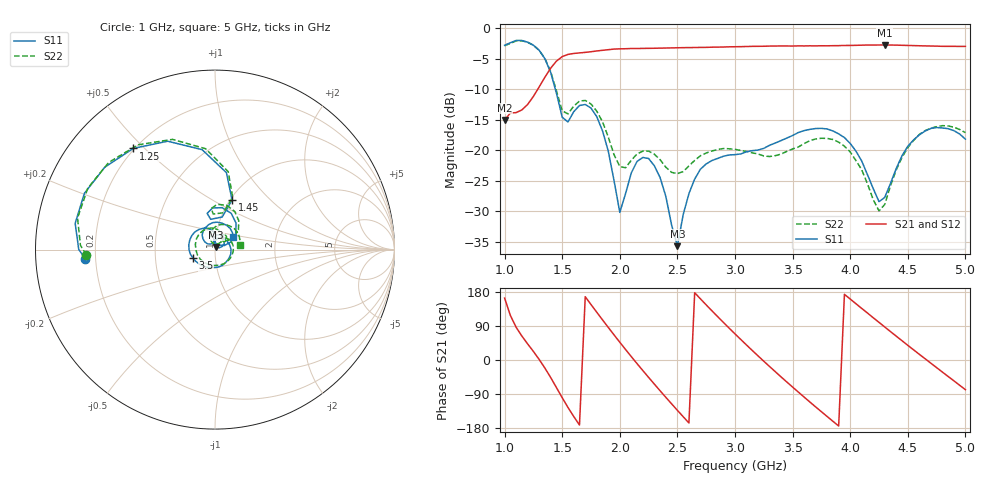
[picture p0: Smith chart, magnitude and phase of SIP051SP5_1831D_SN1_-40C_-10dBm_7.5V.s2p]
# GHz  S  dB  R  50
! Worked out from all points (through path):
!   81 points, 1 GHz to 5 GHz, reference 50 ohm
!   highest |S21| = -2.76 dB at 4.3 GHz (marker M1); lowest = -15.0 dB at 1 GHz (marker M2)
!   lowest |S11| = -35.7 dB at 2.5 GHz (marker M3), VSWR 1.03, Z = 50.6 + j1.55 ohm
!   |S11| at or under -10 dB: 1.44 GHz to end of sweep
!   |S22| runs from -29.9 to -2.1 dB; largest |S21 - S12| = 0.0026
!   S11 on the Smith chart (normalised r, x): 1 GHz: 0.16, -0.04; 1.25 GHz: 0.20, +0.46; 1.45 GHz: 1.02, +0.62; 3.5 GHz: 0.78, -0.07; 5 GHz: 1.21, +0.17
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1  -2.81 -175.9  -15.05 163.3  -15.04 163.5  -2.88 -177.6
1.15  -2.02 156.6  -13.39 63.0  -13.39 63.1  -2.08 154.2
1.25  -2.80 128.9  -11.18 22.6  -11.18 22.5  -2.80 126.3
1.45  -10.67 71.1  -5.40 -72.8  -5.39 -72.8  -10.26 71.2
1.55  -15.37 98.1  -4.30 -125.2  -4.30 -125.1  -14.05 92.8
1.7  -12.51 80.3  -3.97 167.0  -3.97 167.0  -11.85 75.3
1.9  -20.16 25.6  -3.53 86.0  -3.51 86.0  -17.85 33.5
2  -30.19 57.9  -3.39 46.9  -3.38 46.7  -22.66 46.4
2.1  -23.71 96.7  -3.34 8.9  -3.34 8.9  -21.64 66.1
2.35  -24.49 31.9  -3.28 -81.3  -3.27 -81.2  -21.56 40.2
2.5  -35.72 69.2  -3.22 -132.9  -3.22 -132.8  -23.84 47.2
2.7  -23.10 68.3  -3.16 161.4  -3.15 161.3  -20.91 45.2
2.85  -21.34 17.9  -3.11 114.3  -3.11 114.2  -19.88 23.1
3  -20.72 -32.8  -3.05 68.9  -3.04 68.8  -19.86 -6.0
3.25  -19.70 -105.4  -2.97 -3.2  -2.96 -3.3  -20.94 -74.4
3.5  -17.59 -159.5  -2.93 -71.5  -2.92 -71.5  -19.80 -163.3
3.7  -16.45 159.2  -2.91 -123.7  -2.90 -123.8  -18.16 136.4
4  -18.89 101.8  -2.83 160.9  -2.83 160.9  -20.28 69.0
4.3  -27.73 132.3  -2.76 87.1  -2.77 87.1  -28.89 104.8
4.35  -25.43 142.5  -2.77 74.9  -2.78 74.9  -25.82 114.5
4.65  -16.85 103.8  -2.91 3.4  -2.92 3.2  -16.80 75.5
5  -18.19 34.8  -2.99 -78.2  -2.98 -78.3  -17.12 10.9
